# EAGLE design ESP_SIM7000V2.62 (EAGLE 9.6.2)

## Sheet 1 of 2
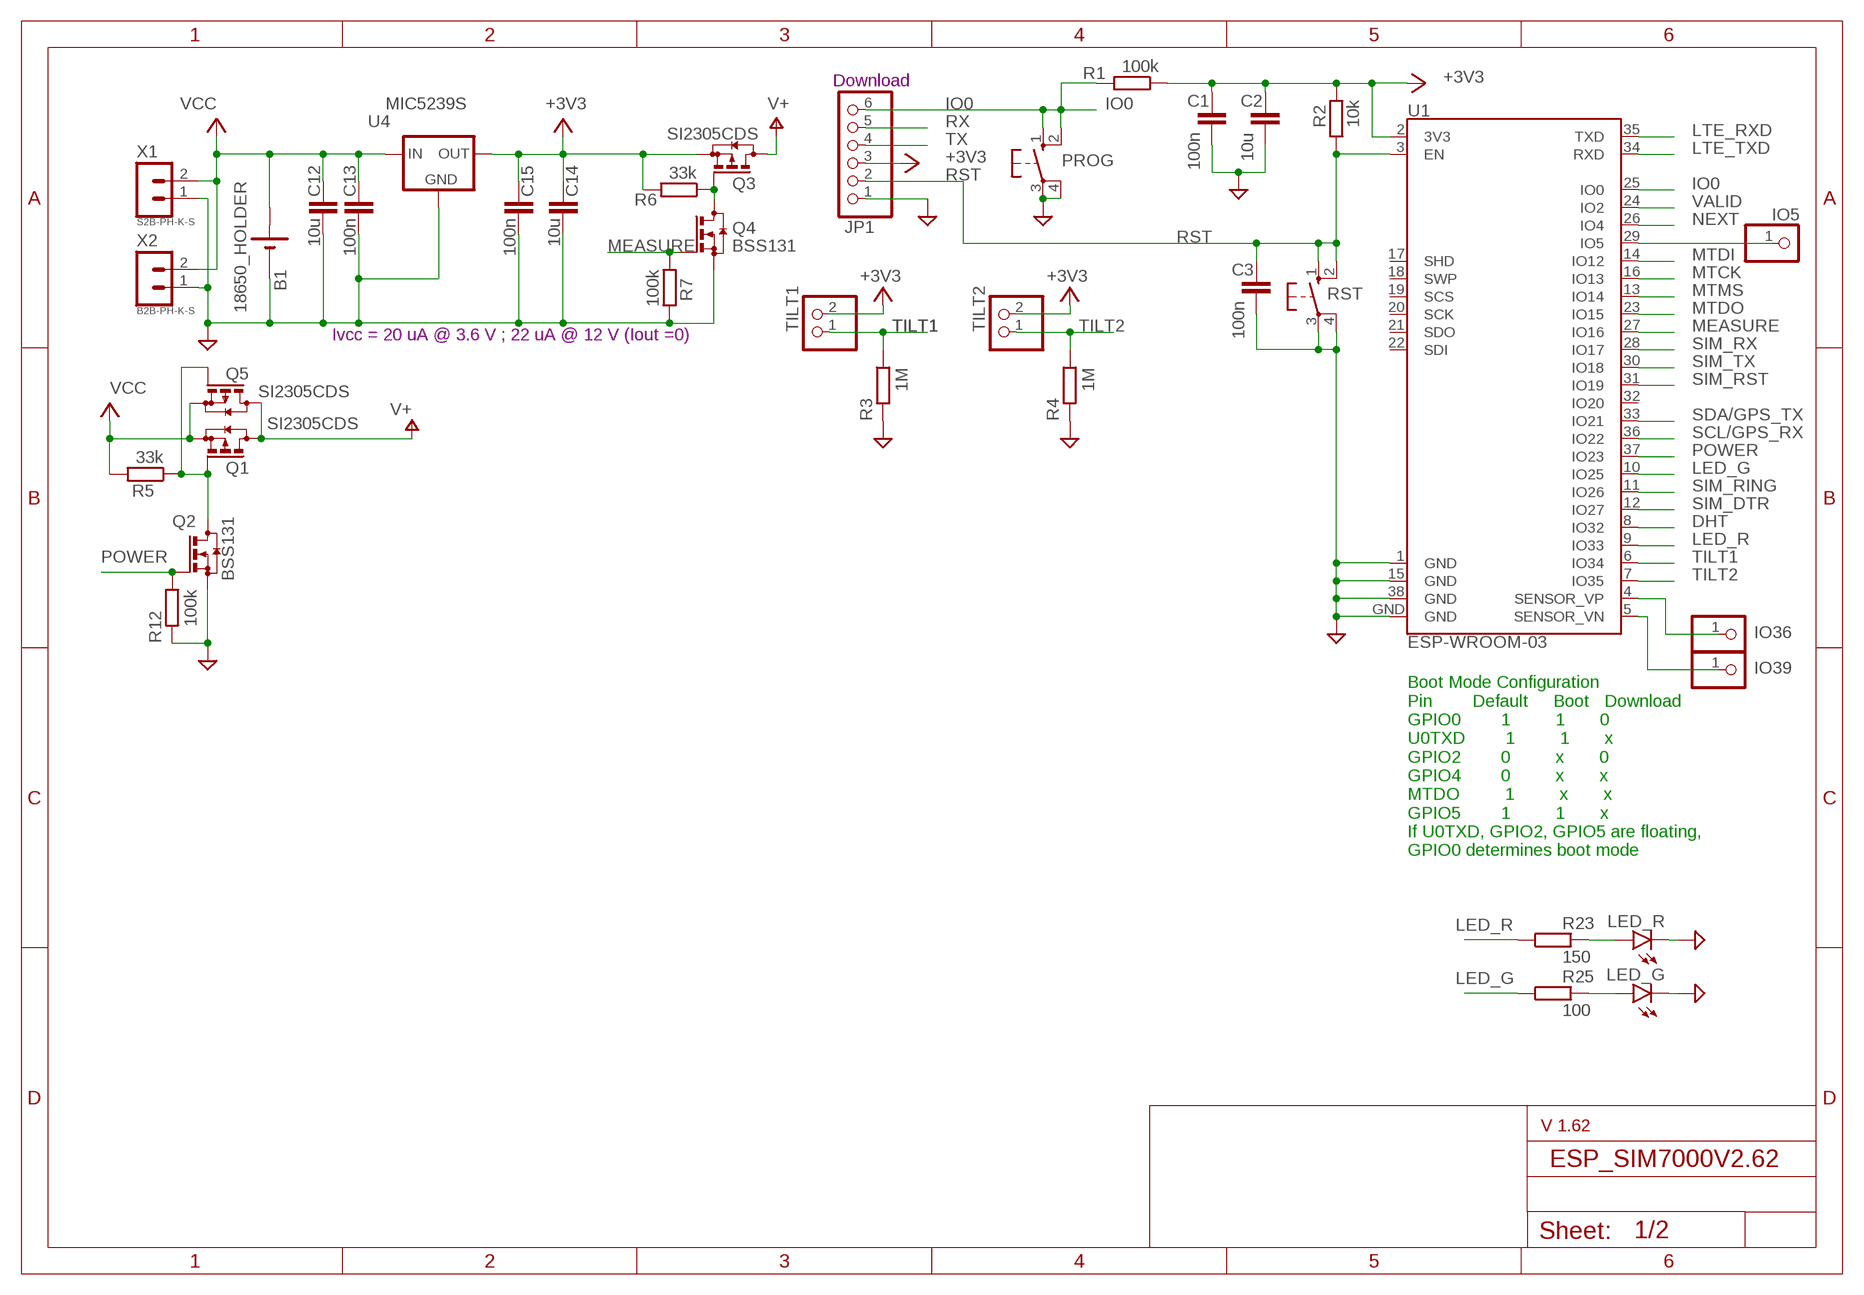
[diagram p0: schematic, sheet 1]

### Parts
B1  18650_HOLDER  [18650]
C1  100n  CC1206  [C1206]
C2  10u  CC1210  [C1210]
C3  100n  CC1206  [C1206]
C12  10u  CC1210  [C1210]
C13  100n  CC1206  [C1206]
C14  10u  CC1210  [C1210]
C15  100n  CC1206  [C1206]
IO5  PINHD-1X1  [1X01]
IO36  PINHD-1X1  [1X01]
IO39  PINHD-1X1  [1X01]
JP1  PINHD-1X6  [1X06]
LED_G  LEDSMT1206  [1206]
LED_R  LEDSMT1206  [1206]
PROG  10-XX  [B3F-10XX]
Q1  SI2305CDS  [SOT23]
Q2  BSS131  [SOT23]
Q3  SI2305CDS  [SOT23]
Q4  BSS131  [SOT23]
Q5  SI2305CDS  [SOT23]
R1  100k  RR1206  [R1206]
R2  10k  RR1206  [R1206]
R3  1M  RR1206  [R1206]
R4  1M  RR1206  [R1206]
R5  33k  RR1206  [R1206]
R6  33k  RR1206  [R1206]
R7  100k  RR1206  [R1206]
R12  100k  RR1206  [R1206]
R23  150  RR1206  [R1206]
R25  100  RR1206  [R1206]
RST  10-XX  [B3F-10XX]
TILT1  PINHD-1X2  [1X02]
TILT2  PINHD-1X2  [1X02]
U1  ESP-WROOM-03  [ESP-WROOM-03]
U4  MIC5239S  [SOT223]
X1  S2B-PH-K-S  [S2B-PH-K-S]
X2  B2B-PH-K-S  [B2B-PH-K-S]

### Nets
+3V3: C1.1 C2.1 C14.1 C15.1 JP1.3 Q3.2(S) R1.1 R2.2 R6.2 TILT1.2 TILT2.2 U1.2(3V3) U4.3(OUT)
DHT: U1.8(IO32)
GND: B1.- C1.2 C2.2 C3.2 C12.2 C13.2 C14.2 C15.2 JP1.1 LED_G.C LED_R.C PROG.3(P) PROG.4(P1) Q2.2(S) Q4.2(S) R3.2 R4.2 R7.2 R12.2 RST.3(P) RST.4(P1) U1.1(GND) U1.15(GND) U1.38(GND) U1.GND U4.2(GND) U4.4(GND) X1.1 X2.1 ; also sheet 2
IO0: JP1.6 PROG.1(S) PROG.2(S1) R1.2 U1.25(IO0)
IO36: IO36.1 U1.4(SENSOR_VP)
IO39: IO39.1 U1.5(SENSOR_VN)
LED_G: R25.1 U1.10(IO25)
LED_R: R23.1 U1.9(IO33) ; also sheet 2
LTE_RXD: U1.35(TXD) ; also sheet 2
LTE_TXD: U1.34(RXD) ; also sheet 2
MEASURE: Q4.1(G) R7.1 U1.27(IO16)
MTCK: U1.16(IO13)
MTDI: U1.14(IO12)
MTDO: U1.23(IO15)
MTMS: U1.13(IO14)
N$1: Q1.1(G) Q2.3(D) Q5.1(G) R5.1
N$2: Q3.1(G) Q4.3(D) R6.1
N$7: LED_R.A R23.2
N$8: LED_G.A R25.2
N$17: IO5.1 U1.29(IO5)
NEXT: U1.26(IO4)
POWER: Q2.1(G) R12.1 U1.37(IO23)
RST: C3.1 JP1.2 R2.1 RST.1(S) RST.2(S1) U1.3(EN)
RX: JP1.5
SCL/GPS_RX: U1.36(IO22)
SDA/GPS_TX: U1.33(IO21)
SIM_DTR: U1.12(IO27)
SIM_RING: U1.11(IO26)
SIM_RST: U1.31(IO19)
SIM_RX: U1.28(IO17)
SIM_TX: U1.30(IO18)
TILT1: R3.1 TILT1.1 U1.6(IO34)
TILT2: R4.1 TILT2.1 U1.7(IO35)
TX: JP1.4
V+: Q1.3(D) Q3.3(D) Q5.3(D)
VALID: U1.24(IO2)
VCC: B1.+ C12.1 C13.1 Q1.2(S) Q5.2(S) R5.2 U4.1(IN) X1.2 X2.2
Unconnected: U1.17(SHD) U1.18(SWP) U1.19(SCS) U1.20(SCK) U1.21(SDO) U1.22(SDI) U1.32(IO20)

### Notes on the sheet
- Download
- Ivcc = 20 uA @ 3.6 V ; 22 uA @ 12 V (Iout =0)
- Boot Mode Configuration
  Pin        Default     Boot   Download
  GPIO0        1         1       0
  U0TXD        1         1       x
  GPIO2        0         x       0
  GPIO4        0         x       x
  MTDO         1         x       x
  GPIO5        1         1       x
  If U0TXD, GPIO2, GPIO5 are floating, 
  GPIO0 determines boot mode
- V 1.62

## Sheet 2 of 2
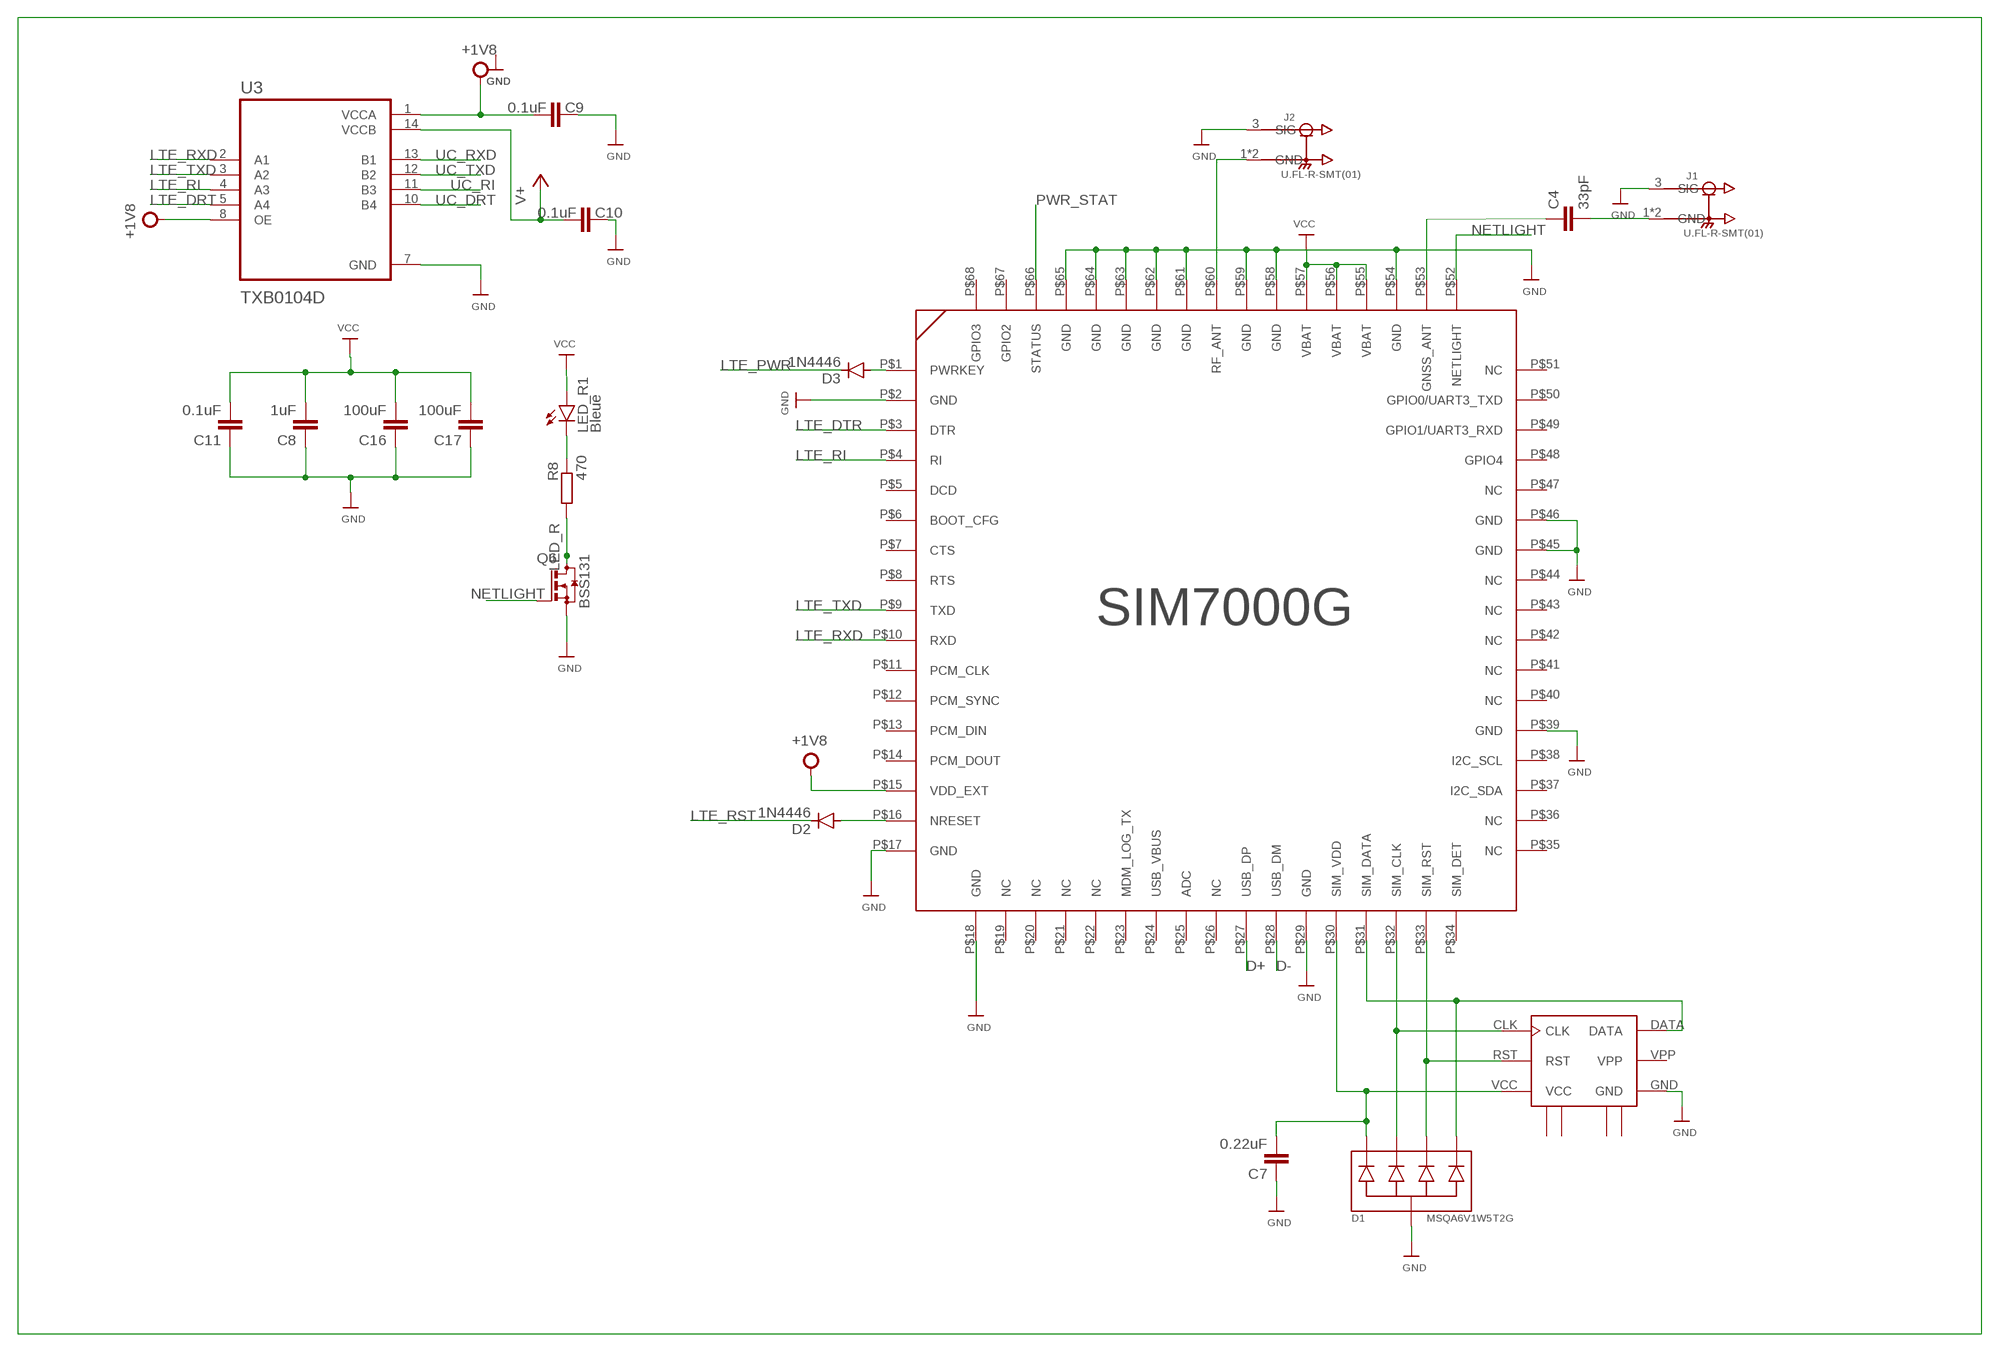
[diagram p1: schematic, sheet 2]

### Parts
C4  33pF  C-EU025-024X044  [C025-024X044]
C7  0.22uF  C-EU025-024X044  [C025-024X044]
C8  1uF  C-EU025-024X044  [C025-024X044]
C9  0.1uF  CC1210  [C1210]
C10  0.1uF  CC1210  [C1210]
C11  0.1uF  C-EU025-024X044  [C025-024X044]
C16  100uF  C-EU025-024X044  [C025-024X044]
C17  100uF  C-EU025-024X044  [C025-024X044]
D1  MSQA6V1W5T2G  [SC88A]
D2  1N4446  [DO35-10]
D3  1N4446  [DO35-10]
J1  U.FL-R-SMT(01)  [HRS_U.FL-R-SMT(01)]
J2  U.FL-R-SMT(01)  [HRS_U.FL-R-SMT(01)]
LED_R1  Bleue  LEDSMT1206  [1206]
Q6  BSS131  [SOT23]
R8  470  RR1206  [R1206]
U3  TXB0104D  [SOIC127P600X175-14N]
U$1  SIM7000G  [SIM7000G]
U$2  SCU-W0822XR-06  [SCU-W0822XR-06]

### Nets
+1V8: C9.2 U3.1(VCCA) U3.8(OE) U$1.P$15(VDD_EXT)
+5V: C10.2 U3.14(VCCB) ; supply symbol labelled V+
D+: U$1.P$27(USB_DP)
D-: U$1.P$28(USB_DM)
GND: C7.1 C8.1 C9.1 C10.1 C11.1 C16.1 C17.1 D1.2 J1.3(SIG) J2.3(SIG) Q6.2(S) U3.7(GND) U$1.P$2(GND) U$1.P$17(GND) U$1.P$18(GND) U$1.P$29(GND) U$1.P$39(GND) U$1.P$45(GND) U$1.P$46(GND) U$1.P$54(GND) U$1.P$55(VBAT) U$1.P$56(VBAT) U$1.P$57(VBAT) U$1.P$58(GND) U$1.P$59(GND) U$1.P$61(GND) U$1.P$62(GND) U$1.P$63(GND) U$1.P$64(GND) U$1.P$65(GND) U$2.GND ; supply symbol labelled VCC ; also sheet 1
LED_R: Q6.3(D) R8.1 ; also sheet 1
LTE_DRT: U3.5(A4)
LTE_DTR: U$1.P$3(DTR)
LTE_PWR: D3.C
LTE_RI: U3.4(A3) U$1.P$4(RI)
LTE_RST: D2.C
LTE_RXD: U3.2(A1) U$1.P$10(RXD) ; also sheet 1
LTE_TXD: U3.3(A2) U$1.P$9(TXD) ; also sheet 1
N$3: J2.1(GND) J2.2(GND) U$1.P$60(RF_ANT)
N$4: C4.2 J1.1(GND) J1.2(GND)
N$5: C4.1 U$1.P$53(GNSS_ANT)
N$6: D2.A U$1.P$16(NRESET)
N$10: LED_R1.C R8.2
N$11: C7.2 D1.1 U$1.P$30(SIM_VDD) U$2.VCC
N$12: D1.5 U$1.P$31(SIM_DATA) U$2.DATA
N$13: D1.3 U$1.P$32(SIM_CLK) U$2.CLK
N$14: D1.4 U$1.P$33(SIM_RST) U$2.RST
N$15: LED_R1.A
N$18: D3.A U$1.P$1(PWRKEY)
N$19: C8.2 C11.2 C16.2 C17.2
NETLIGHT: Q6.1(G) U$1.P$52(NETLIGHT)
PWR_STAT: U$1.P$66(STATUS)
UC_DRT: U3.10(B4)
UC_RI: U3.11(B3)
UC_RXD: U3.13(B1)
UC_TXD: U3.12(B2)
Unconnected: U$1.P$5(DCD) U$1.P$6(BOOT_CFG) U$1.P$7(CTS) U$1.P$8(RTS) U$1.P$11(PCM_CLK) U$1.P$12(PCM_SYNC) U$1.P$13(PCM_DIN) U$1.P$14(PCM_DOUT) U$1.P$19(NC) U$1.P$20(NC) U$1.P$21(NC) U$1.P$22(NC) U$1.P$23(MDM_LOG_TX) U$1.P$24(USB_VBUS) U$1.P$25(ADC) U$1.P$26(NC) U$1.P$34(SIM_DET) U$1.P$35(NC) U$1.P$36(NC) U$1.P$37(I2C_SDA) U$1.P$38(I2C_SCL) U$1.P$40(NC) U$1.P$41(NC) U$1.P$42(NC) U$1.P$43(NC) U$1.P$44(NC) U$1.P$47(NC) U$1.P$48(GPIO4) U$1.P$49(GPIO1/UART3_RXD) U$1.P$50(GPIO0/UART3_TXD) U$1.P$51(NC) U$1.P$67(GPIO2) U$1.P$68(GPIO3)

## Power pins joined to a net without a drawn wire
GND1: U$2.GND_1(GND1)
GND2: U$2.GND_2(GND2)
GND3: U$2.GND_3(GND3)
GND4: U$2.GND_4(GND4)
VPP: U$2.VPP

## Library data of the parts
B1 = battery_bms:18650_HOLDER: 18650 holder
C1-C3 C9 C10 C12-C15 = eagle-ltspice:C: CAPACITOR, European symbol; SPICEMODEL: NONE; SPICEPREFIX: C
C4 C7 C8 C11 C16 C17 = rcl:C-EU: CAPACITOR, European symbol; SPICEPREFIX: C
D1 = MSQA6V1W5T2G:MSQA6V1W5T2G: ESD Protection Diode Array Check availability; AVAILABILITY: In Stock; CHECK_PRICES: https://www.snapeda.com/parts/MSQA6V1W5T2G/Onsemi/view-part/?ref=eda; DESCRIPTION: Clamp Ipp Tvs Diode Surface Mount SC-88A (SC-70-5/SOT-353); MF: onsemi; MP: MSQA6V1W5T2G; PACKAGE: SC-88A-5 ON Semiconductor; PRICE: None; PURCHASE-URL: https://www.snapeda.com/api/url_track_click_mouser/?unipart_id=7122110&manufacturer=onsemi&part_name=MSQA6V1W5T2G&search_term=msqa6v1w5t2g; SNAPEDA_LINK: https://www.snapeda.com/parts/MSQA6V1W5T2G/Onsemi/view-part/?ref=snap
D2 D3 = diode:1N4446: DIODE
IO5 IO36 IO39 = pinhead:PINHD-1X1: PIN HEADER
J1 J2 = U.FL-R-SMT_01_:U.FL-R-SMT(01): U.FL Series 6 Ghz 50 Ohm Ultra-small SMT Coaxial Cable Receptacle Check availability; AVAILABILITY: In Stock; CHECK_PRICES: https://www.snapeda.com/parts/U.FL-R-SMT(01)/Hirose+Electric+Co+Ltd/view-part/?ref=eda; DESCRIPTION: U.FL (UMCC) Connector Receptacle, Male Pin 50Ohm Surface Mount Solder. RF Connectors / Coaxial Connectors; MF: Hirose; MP: U.FL-R-SMT(01); PACKAGE: None; PRICE: None; PURCHASE-URL: https://www.snapeda.com/api/url_track_click_mouser/?unipart_id=49572&manufacturer=Hirose&part_name=U.FL-R-SMT(01)&search_term=None; SNAPEDA_LINK: https://www.snapeda.com/parts/U.FL-R-SMT(01)/Hirose+Electric+Co+Ltd/view-part/?ref=snap
JP1 = pinhead:PINHD-1X6: PIN HEADER
LED_G LED_R LED_R1 = led:LED: LED
PROG RST = switch-omron:10-XX: OMRON SWITCH; MPN: B3F-1000; OC_FARNELL: 176432; OC_NEWARK: 36M3542
Q1 Q3 Q5 = transistor-small-signal-perso:SI2305CDS: P-CHANNEL MOS FET
Q2 Q4 Q6 = transistor-small-signal-perso:BSS131: N-CHANNEL MOS FET
R1-R8 R12 R23 R25 = eagle-ltspice:R: RESISTOR, European symbol; SPICEMODEL: NONE; SPICEPREFIX: R
TILT1 TILT2 = pinhead:PINHD-1X2: PIN HEADER
U1 = esp32-sparkfun (1):ESP-WROOM-03; OC_FARNELL: unknown
U3 = TXB0104D:TXB0104D; CHECK_PRICES: https://www.snapeda.com/parts/TXB0104D/Texas+Instruments/view-part/?ref=eda; DESCRIPTION: 4-Bit Bidirectional Voltage-Level Shifter with Auto Direction Sensing and +/-15 kV ESD Protect; MF: Texas Instruments; MP: TXB0104D; PACKAGE: SOIC-14 Texas Instruments; PURCHASE-URL: https://www.snapeda.com/api/url_track_click_mouser/?unipart_id=44550&manufacturer=Texas Instruments&part_name=TXB0104D&search_term=txb0104; RS_COMPONENTS_7092778P_PURCHASE_URL: https://www.snapeda.com/api/url_track_click/https%253A//uk.rs-online.com/web/p/translator-ics/7092778p//%253Futm_campaign%253Dbuynow%2526utm_medium%253Daggregator%2526utm_source%253Dsnapeda%2526cm_mmc%253Daff-_-uk-_-snapeda-_-7092778P/?unipart_id=44550&manufacturer=Texas Instruments&part_name=TXB0104D&search_term=txb0104; RS_COMPONENTS_7092778_PURCHASE_URL: https://www.snapeda.com/api/url_track_click/https%253A//uk.rs-online.com/web/p/translator-ics/7092778//%253Futm_campaign%253Dbuynow%2526utm_medium%253Daggregator%2526utm_source%253Dsnapeda%2526cm_mmc%253Daff-_-uk-_-snapeda-_-7092778/?unipart_id=44550&manufacturer=Texas Instruments&part_name=TXB0104D&search_term=txb0104; RS_COMPONENTS_9236790_PURCHASE_URL: https://www.snapeda.com/api/url_track_click/https%253A//uk.rs-online.com/web/p/translator-ics/9236790//%253Futm_campaign%253Dbuynow%2526utm_medium%253Daggregator%2526utm_source%253Dsnapeda%2526cm_mmc%253Daff-_-uk-_-snapeda-_-9236790/?unipart_id=44550&manufacturer=Texas Instruments&part_name=TXB0104D&search_term=txb0104; SNAPEDA_LINK: https://www.snapeda.com/parts/TXB0104D/Texas+Instruments/view-part/?ref=snap
U4 = micrel:MIC5239S: LDO REGULATOR
U$1 = SIM7000G:SIM7000G; CHECK_PRICES: https://www.snapeda.com/parts/SIM7000G/SIMCom/view-part/?ref=eda; DESCRIPTION: 802.15.4 Cat-M, Cat-NB, EDGE, GPRS, LPWA Transceiver Module 850MHz, 900MHz, 1.8GHz, 1.9GHz Antenna Not Included Surface Mount; MF: SIMCom Wireless Solutions Limited; MP: SIM7000G; PACKAGE: None; PURCHASE-URL: https://www.snapeda.com/api/url_track_click_mouser/?unipart_id=12130268&manufacturer=SIMCom Wireless Solutions Limited&part_name=SIM7000G&search_term=sim7000g; SNAPEDA_LINK: https://www.snapeda.com/parts/SIM7000G/SIMCom/view-part/?ref=snap
U$2 = con-sim:SCU-W0822XR-06
X1 = con-JST PH:S2B-PH: JST PH series header 2.00mm pitch disconnectable crimp style connectors, horizontal (side entry type), 2 pins
X2 = con-JST PH:B2B-PH: JST PH series header 2.00mm pitch disconnectable crimp style connectors, vertical (side entry type), 2 pins

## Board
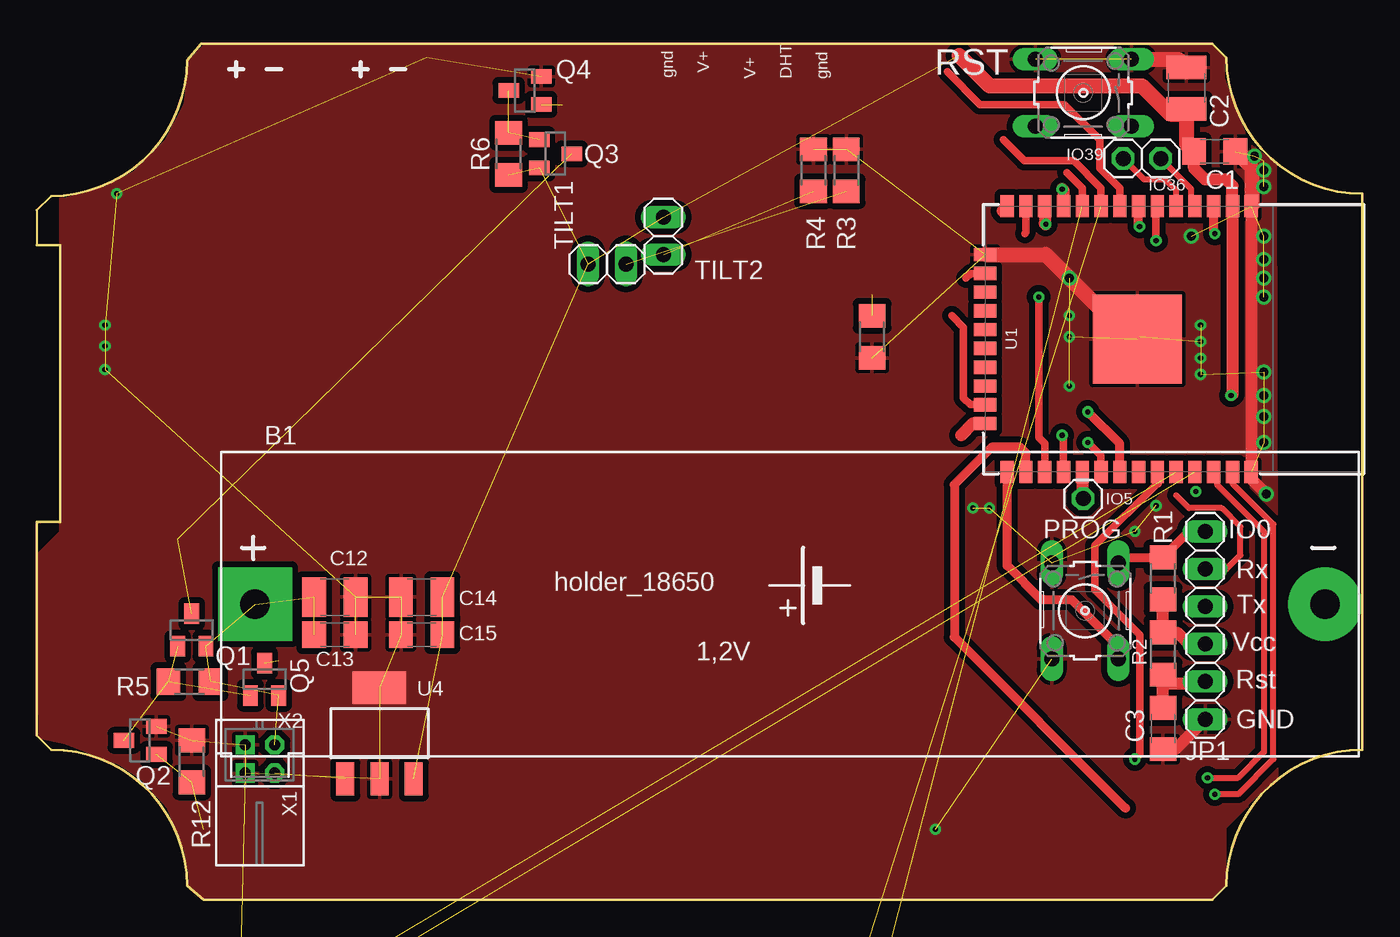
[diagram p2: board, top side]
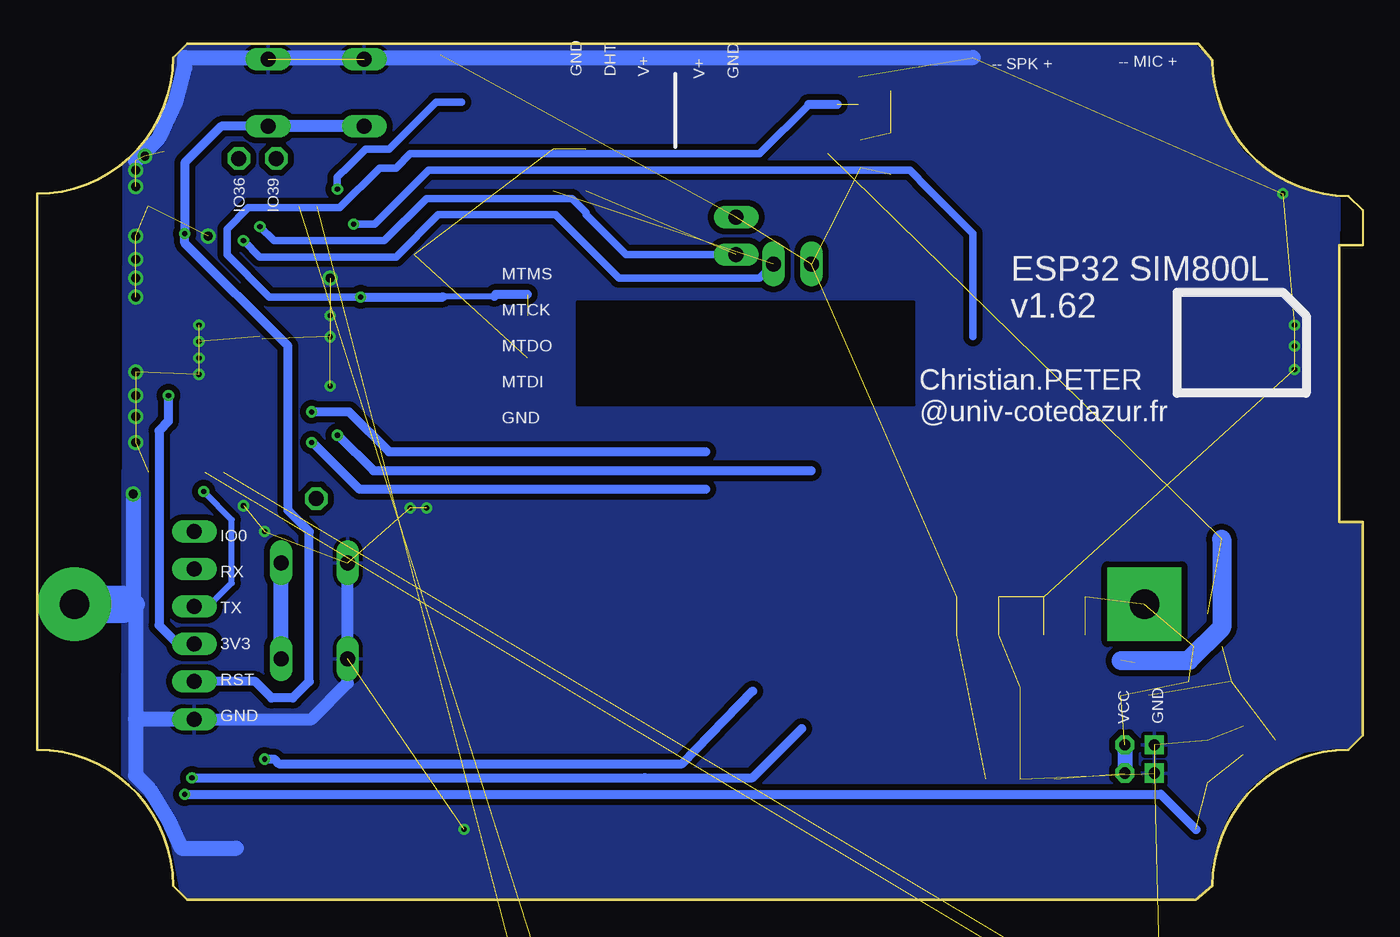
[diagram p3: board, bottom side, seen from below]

Size 89.69 x 57.94 mm. Coordinates in mm from the lower left corner, seen from the top.
Outline: 0.95,10.16 arc-90 10.16,0.95
Outline: 10.16,0.95 11.27,0 79.53,0 80.49,0.95 arc-90 89.69,10.16 89.69,47.78 arc-90 80.49,56.99 79.53,57.94 11.11,57.94 10.16,56.83 arc-90 0.95,47.62 0,46.67 0,44.29 1.59,44.29 1.59,25.56 0,25.56 0,11.11 0.95,10.16
Outline: 0.95,10.16 arc-90 10.16,0.95
Copper layers (1*16): Top 0.035mm / dielectric 1.5mm / Bottom 0.035mm
Design rules "default *": minimum track width 6mil, minimum drill 0.35mm, track to track 6mil, track to pad 6mil, pad to pad 6mil, via to via 6mil, smd to smd 6mil, copper to edge 0mil, drill to drill 6mil, minimum pad ring 10mil, minimum via ring 8mil, stop-mask expansion 4mil, vias tented up to drill 0mil, thermal gap 10mil

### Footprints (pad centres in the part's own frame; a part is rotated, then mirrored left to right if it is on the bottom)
18650 = drill 2 pad 5 square: + -36.2,0 | drill 2 pad 5: - 36.2,0
C1206 = smd 1.6 x 1.8: 1 -1.4,0; 2 1.4,0
C1210 = smd 1.6 x 2.7: 1 -1.4,0; 2 1.4,0
C025-024X044 = drill 0.813 octagon: 1 -1.27,0; 2 1.27,0
SC88A = smd 0.5 x 0.4: 1 0,0.65; 2 0,0; 3 0,-0.65; 4 1.9,-0.65; 5 1.9,0.65
DO35-10 = drill 0.813 long: A 5.08,0; C -5.08,0
1X01 = drill 1.016 octagon: 1 0,0
HRS_U.FL-R-SMT(01) = smd 1.1 x 2.25: 1 -1.475,0; 2 1.475,0 | smd 1.05 x 1.1: 3 0,-1.55
1X06 = drill 1.016 long: 1 -6.35,0; 2 -3.81,0; 3 -1.27,0; 4 1.27,0; 5 3.81,0; 6 6.35,0
1206 = smd 1.6 x 1.803: A -1.422,0; C 1.422,0
B3F-10XX = drill 1.016 long: 1 -3.251,2.261; 2 3.251,2.261; 3 -3.251,-2.261; 4 3.251,-2.261
SOT23 = smd 1 x 1.4: 1 -0.95,-1.1; 2 0.95,-1.1; 3 0,1.1
R1206 = smd 1.6 x 1.803: 1 -1.422,0; 2 1.422,0
1X02 = drill 1.016 long: 1 -1.27,0; 2 1.27,0
ESP-WROOM-03 = smd 0.9 x 1.5: 1 7.7,9; 2 6.43,9; 3 5.16,9; 4 3.89,9; 5 2.62,9; 6 1.35,9; 7 0.08,9; 8 -1.19,9; 9 -2.46,9; 10 -3.73,9; 11 -5,9; 12 -6.27,9; 13 -7.54,9; 14 -8.81,9; 25 -8.81,-9; 26 -7.54,-9; 27 -6.27,-9; 28 -5,-9; 29 -3.73,-9; 30 -2.46,-9; 31 -1.19,-9; 32 0.08,-9; 33 1.35,-9; 34 2.62,-9; 35 3.89,-9; 36 5.16,-9; 37 6.43,-9; 38 7.7,-9 | smd 1.5 x 0.9: 15 -10.3,5.715; 16 -10.3,4.445; 17 -10.3,3.175; 18 -10.3,1.905; 19 -10.3,0.635; 20 -10.3,-0.635; 21 -10.3,-1.905; 22 -10.3,-3.175; 23 -10.3,-4.445; 24 -10.3,-5.715 | smd 6 x 6: GND 0,0
SOIC127P600X175-14N = smd 1.97 x 0.6: 1 -2.475,3.81; 2 -2.475,2.54; 3 -2.475,1.27; 4 -2.475,0; 5 -2.475,-1.27; 6 -2.475,-2.54; 7 -2.475,-3.81; 8 2.475,-3.81; 9 2.475,-2.54; 10 2.475,-1.27; 11 2.475,0; 12 2.475,1.27; 13 2.475,2.54; 14 2.475,3.81
SOT223 = smd 1.219 x 2.235: 1 -2.311,-3.099; 2 0,-3.099; 3 2.311,-3.099 | smd 3.6 x 2.2: 4 0,3.099
SIM7000G = smd 2 x 0.5: P$1 -12,8; P$2 -12,7; P$3 -12,6; P$4 -12,5; P$5 -12,4; P$6 -12,3; P$7 -12,2; P$8 -12,1; P$9 -12,0; P$10 -12,-1; P$11 -12,-2; P$12 -12,-3; P$13 -12,-4; P$14 -12,-5; P$15 -12,-6; P$16 -12,-7; P$17 -12,-8; P$35 12,-8; P$36 12,-7; P$37 12,-6; P$38 12,-5; P$39 12,-4; P$40 12,-3; P$41 12,-2; P$42 12,-1; P$43 12,0; P$44 12,1; P$45 12,2; P$46 12,3; P$47 12,4; P$48 12,5; P$49 12,6; P$50 12,7; P$51 12,8 | smd 0.5 x 2: P$18 -8,-12; P$19 -7,-12; P$20 -6,-12; P$21 -5,-12; P$22 -4,-12; P$23 -3,-12; P$24 -2,-12; P$25 -1,-12; P$26 0,-12; P$27 1,-12; P$28 2,-12; P$29 3,-12; P$30 4,-12; P$31 5,-12; P$32 6,-12; P$33 7,-12; P$34 8,-12; P$52 8,12; P$53 7,12; P$54 6,12; P$55 5,12; P$56 4,12; P$57 3,12; P$58 2,12; P$59 1,12; P$60 0,12; P$61 -1,12; P$62 -2,12; P$63 -3,12; P$64 -4,12; P$65 -5,12; P$66 -6,12; P$67 -7,12; P$68 -8,12
SCU-W0822XR-06 = smd 1.65 x 1.2: CLK -4.42,1.36; DATA 4.43,1.35; GND 4.43,-3.73; RST -4.42,-1.18; VCC -4.42,-3.72; VPP 4.43,-1.19 | smd 2.8 x 2.05: GND_1 2.05,-7.32; GND_2 -4.57,-7.32; GND_3 2.05,7.32; GND_4 -4.57,7.32
S2B-PH-K-S = drill 0.75 pad 1.3 square: 1 1,0 | drill 0.75 pad 1.3 octagon: 2 -1,0
B2B-PH-K-S = drill 0.75 pad 1.3 square: 1 1,0 | drill 0.75 pad 1.3 octagon: 2 -1,0

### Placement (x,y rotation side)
B1  50.96,20 0 top
C1  79.69,50.64 0 top
C2  77.79,54.93 90 top
C3  76.2,11.59 270 top
C4  not placed on the board
C7  not placed on the board
C8  not placed on the board
C9  not placed on the board
C10  not placed on the board
C11  not placed on the board
C12  20.16,20.48 0 top
C13  20.16,17.94 0 top
C14  26.04,20.48 180 top
C15  26.04,17.94 180 top
C16  not placed on the board
C17  not placed on the board
D1  not placed on the board
D2  not placed on the board
D3  not placed on the board
IO5  70.8,27.15 0 top
IO36  76.04,50.16 0 top
IO39  73.5,50.16 90 top
J1  not placed on the board
J2  not placed on the board
JP1  79.06,18.57 90 top
LED_G  not placed on the board
LED_R  not placed on the board
LED_R1  not placed on the board
PROG  70.93,19.56 270 top
Q1  10.48,18.26 0 top
Q2  6.98,10.79 90 top
Q3  35.08,50.48 270 top
Q4  33.02,54.77 90 top
Q5  15.4,14.92 0 top
Q6  not placed on the board
R1  76.2,21.75 90 top
R2  76.2,16.67 90 top
R3  54.77,49.37 90 top
R4  52.55,49.37 90 top
R5  10.32,14.76 0 top
R6  31.91,50.48 270 top
R7  56.52,38.1 270 top
R8  not placed on the board
R12  10.48,9.37 90 top
R23  not placed on the board
R25  not placed on the board
RST  70.8,54.61 180 top
TILT1  38.58,43.02 180 top
TILT2  42.39,44.93 90 top
U1  74.46,37.95 0 top
U3  not placed on the board
U4  23.18,11.27 0 top
U$1  not placed on the board
U$2  not placed on the board
X1  15.08,8.57 180 top
X2  15.08,10.48 180 top

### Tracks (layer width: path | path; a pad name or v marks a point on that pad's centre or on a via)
+1V8  (3 unrouted)
+3V3  (via drill 0.35)  (7 unrouted)
  Top 0.813: JP1.3 77.95,17.3 77.16,18.09 R2.2 R1.1 | C1.1 78.29,49.5 79.06,48.74 80.49,48.74 80.89,48.33 U1.2 80.89,34.22 v80.8,34.13
  Top 1.016: 62.39,57.15 64.45,55.09 74.77,55.09 76.68,53.18 77.44,53.18 C2.1 77.79,51.15 C1.1
  Bottom 0.61: JP1.3 80.17,17.3 81.44,18.57 81.44,31.75 80.8,32.38 v80.8,34.13
+5V  (1 unrouted)
DHT
  Top 0.508: U1.8 73.27,48.17 71.91,49.53 71.91,51.44 69.53,53.82 63.82,53.82 61.6,56.04
GND  (via drill 0.35, 0.6)  (79 unrouted)
  Top 0.61: U1.GND 74.62,38.1
  Top 0.813: v83.19,27.46 82.16,28.49 U1.38 U1.1 82.21,46.99 82.23,46.99 | C3.2 77.02,10.19 JP1.1
  Top 1.016: U1.15 68.26,43.66 73.82,38.1 74.31,38.1 U1.GND | 82.23,46.99 82.23,49.5 C1.2 | RST.3 77.24,56.87 C2.2
  Bottom 0.813: RST.3 74.17,56.99 | JP1.1 71.12,12.22 68.67,14.67 PROG.4 PROG.3
  Bottom 1.016: v83.19,27.46 83.19,20 | 83.03,20 83.03,12.22 | 83.03,12.22 83.03,8.41 82.07,7.46 80.8,5.4 79.94,3.49 76.2,3.49 | 83.03,50.01 81.44,51.59 80.33,53.97 79.69,56.3 79.69,56.99 67.67,56.99 RST.4 67.43,56.99 53.18,56.99 42.55,56.99 26.35,56.99 | JP1.1 83.03,12.22
  Bottom 1.27: 83.98,20 83.19,20 83.03,20
  Bottom 2.54: B1.- 83.98,20
  other vias: 83.03,43.34 83.03,35.72 83.03,42.07 83.03,30.96 83.03,44.93 83.03,40.8 83.03,34.13 83.03,32.7 69.85,42.07 4.6,35.88 4.6,37.47 4.6,38.89 69.85,39.53 69.85,38.1 69.85,34.77 5.4,47.78 64.45,26.51 63.34,26.51 60.8,4.76 83.03,48.26 78.11,44.93 82.39,50.32 83.03,49.37 74.3,24.92 75.72,26.67 78.74,38.89 78.74,37.78 78.74,36.67 78.74,35.56
  pour Top (isolate 0.406): 11.27,0 10.32,0.79 10.32,1.75 10,3.49 8.89,6.19 6.98,8.25 5.56,9.21 1.94,10.6 0.18,10.95 0.07,23.4 1.59,24.92 1.59,47.47 1.9,47.47 4.76,48.26 6.51,49.21 8.73,51.44 10,53.82 10.32,56.83 11.27,57.79 79.53,57.79 80.33,56.99 80.33,55.56 81.98,51.18 83.82,49.81 83.93,8.33 81.9,6.43 81.9,6.33 80.41,4.85 80.41,1.04 79.38,0
  pour Bottom (isolate 0.406): 11.27,0 10.32,0.95 10.32,2.06 9.84,4.13 9.05,5.87 7.78,7.46 6.35,8.73 3.97,10 1.75,10.32 0.95,10.32 0.16,11.11 0,25.4 1.75,25.4 1.59,47.47 3.65,47.94 5.4,48.58 6.83,49.53 8.1,50.64 8.89,51.75 10,54.13 10.32,56.83 11.27,57.79 79.53,57.79 80.33,56.99 80.33,52.41 83.82,49.81 83.93,8.45 81.21,5.89 81.21,5.32 80.79,4.91 79.98,0.61 79.38,0
  cutout Bottom: 30.32,40.48 53.18,40.48 53.18,33.5 30.32,33.5
IO0
  Top 0.61: 65.56,28.86 U1.25 65.65,22.61 67.95,20.32 70.01,20.32 73.19,17.14 PROG.2 | PROG.1 73.55,23.17 R1.2 77.95,24.92 JP1.6
  Bottom 1.016: PROG.2 PROG.1
IO36
  Top 0.406: U1.4 78.35,47.38 78.11,47.62 78.11,48.1 IO36.1
IO39
  Top 0.406: U1.5 77.08,48.01 76.36,48.74 74.93,48.74 IO39.1
LED_G  (1 unrouted)
  Top 0.508: 69.69,49.21 70.73,48.17 U1.10
LED_R  (3 unrouted)
  Top 0.508: U1.9 72,48.17 70.17,50.01 66.83,50.01 65.4,51.44
LTE_RI  (1 unrouted)
LTE_RXD  (2 unrouted)
LTE_TXD  (2 unrouted)
MEASURE  (via drill 0.35)  (2 unrouted)
  Top 0.508: U1.27 68.19,30.87 67.79,31.27 v67.79,40.8
  Bottom 0.406: 58.74,40.85 62.18,40.85 62.23,40.8
  Bottom 0.508: 37.46,53.82 40.8,50.48 64.45,50.48 65.41,49.53 66.52,49.53 69.22,46.83 75.41,46.83 76.84,45.4 76.84,43.66 73.98,40.8 v67.79,40.8
  Bottom 0.61: 35.56,53.82 37.46,53.82 | 56.52,40.96 58.63,40.96 58.74,40.85 | v67.79,40.8 62.23,40.8
MTCK
  Top 0.508: U1.16 63.19,42.39 62.87,42.07
MTDI
  Top 0.813: U1.14 65.34,46.63
MTDO
  Top 0.508: U1.23 63.18,33.5 62.71,33.97 62.71,38.73 61.91,39.53
MTMS
  Top 0.508: 66.83,45.08 66.92,45.18 U1.13
N$1  (3 unrouted)
N$2  (2 unrouted)
N$3  (2 unrouted)
N$4  (2 unrouted)
N$5  (1 unrouted)
N$6  (1 unrouted)
N$7  (1 unrouted)
N$8  (1 unrouted)
N$10  (1 unrouted)
N$11  (3 unrouted)
N$12  (2 unrouted)
N$13  (2 unrouted)
N$14  (2 unrouted)
N$17
  Top 0.813: U1.29 70.73,27.21 IO5.1
N$18  (1 unrouted)
N$19  (3 unrouted)
NETLIGHT  (1 unrouted)
NEXT
  Top 0.61: U1.26 66.92,30.23 66.52,30.64 64.61,30.64 62.07,28.1 62.07,17.78 73.66,6.19
POWER  (via drill 0.35)  (2 unrouted)
  Top 0.406: v79.69,7.14 81.28,7.14 83.66,9.53 83.66,25.4 80.89,28.17 U1.37
  Bottom 0.61: v79.69,7.14 13.65,7.14 11.27,4.76
RST  (via drill 0.35)
  Top 0.61: v79.69,45.08 79.62,45.15 U1.3
  Top 0.813: C3.1 76.2,14.6 | 76.2,14.6 R2.1 | JP1.2 78.9,14.6 76.2,14.6
  Bottom 0.61: JP1.2 74.93,14.76 73.82,13.65 72.39,13.65 71.28,14.76 71.28,24.92 72.71,26.35 72.71,37.47 79.69,44.45 v79.69,45.08 79.69,49.89 77.23,52.35 RST.1
  Bottom 0.813: RST.2 RST.1
RX
  Top 0.406: JP1.5 80.49,22.38 81.44,23.34 81.44,25.24 80.17,26.51 77.95,26.51 77.08,27.37
SCL/GPS_RX  (via drill 0.35)
  Top 0.406: v79.22,8.25 81.28,8.25 83.03,10 83.03,24.92 79.85,28.1 79.85,28.72 U1.36
  Bottom 0.61: v79.22,8.25 48.58,8.25 41.28,8.25 37.94,11.59
SDA/GPS_TX  (via drill 0.35)
  Top 0.508: 75.81,28.19 71.6,23.97 71.6,20.96 74.61,17.94 74.61,9.84 v74.3,9.53
  Top 0.61: 75.81,28.63 75.97,28.79 U1.33 75.81,28.19
  Bottom 0.61: v74.3,9.53 73.66,9.53 73.34,9.21 46.04,9.21 41.28,14.13
SIM_DTR  (via drill 0.35)
  Top 0.813: U1.12 68.19,45.79 v68.26,45.72
  Bottom 0.508: 26.35,38.1 26.35,45.08 29.37,48.1 30.64,49.37 63.18,49.37 66.83,45.72 v68.26,45.72
SIM_RING  (via drill 0.35)
  Top 0.813: v69.37,48.1 69.46,48.01 U1.11
  Bottom 0.508: v69.37,48.1 69.37,48.9 68.58,49.69 67.47,50.8 65.88,50.8 62.71,53.97 60.96,53.97
SIM_RST  (via drill 0.35)
  Top 0.61: U1.31 73.27,30.87 v71.12,33.02
  Bottom 0.61: 44.45,30.32 65.88,30.32 68.58,33.02 v71.12,33.02
SIM_RX  (via drill 0.35)
  Top 0.508: U1.28 69.46,31.43 v69.37,31.43
  Bottom 0.61: v69.37,31.43 69.3,31.43 66.92,29.05 37.31,29.05
SIM_TX  (via drill 0.35)
  Top 0.508: U1.30 72,30.07 v71.12,30.96
  Bottom 0.61: 44.45,27.78 67.86,27.78 71.03,30.96 v71.12,30.96
TILT1  (via drill 0.35)  (1 unrouted)
  Top 0.508: v75.72,44.61 75.72,46.86 U1.6
  Bottom 0.508: v75.72,44.61 74.61,43.5 65.41,43.5 62.55,46.36 54.61,46.36 50.32,42.07 40.8,42.07 TILT1.1
TILT2  (via drill 0.35)  (1 unrouted)
  Top 0.61: v74.61,45.56 74.54,45.63 U1.7
  Bottom 0.508: v74.61,45.56 73.66,44.61 66.2,44.61 63.34,47.47 53.5,47.47 52.55,46.51 52.55,46.36 49.85,43.66 TILT2.1
TX  (via drill 0.35)
  Top 0.61: 78.35,27.69 v78.42,27.62
  Bottom 0.406: JP1.4 78.11,19.84 76.52,21.43 76.52,25.72 v78.42,27.62
V+  (3 unrouted)
  Bottom 1.27: 16.35,16.19 11.75,16.19 9.53,18.42 9.53,24.42
VALID
  Top 0.61: 64.01,32.38 U1.24
  Top 0.813: U1.24 63.35,32.23 62.54,31.43
VCC  (7 unrouted)
  Bottom 1.016: X2.2 X1.2

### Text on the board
tNames: gnd / / V+ | V+ / / DHT / / gnd | IO0 | Rx | Tx | Vcc | Rst | GND
bNames: -- MIC + | -- SPK + | V+ / / GND | GND / / DHT / / V+ | IO36 / / IO39 | ESP32 SIM800L / v1.62 | Christian.PETER / @univ-cotedazur.fr | MTMS / / MTCK / / MTDO / / MTDI / / GND | IO0 / / RX / / TX / / 3V3 / / RST / / GND | VCC / / GND

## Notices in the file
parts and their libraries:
micrel: Copyright (C) 2008, Bob Starr
